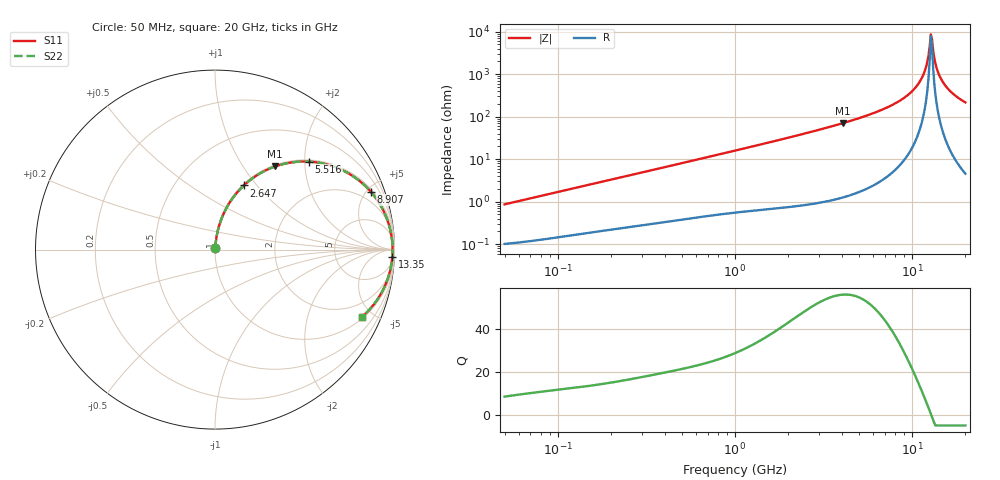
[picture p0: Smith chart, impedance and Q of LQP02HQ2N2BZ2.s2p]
!Murata Part Number: LQP02HQ2N2BZ2
!These Parameters are Measured in Series Mode Connection
!  o--[Z]--o
!Port1  Port2
!  o-------o
!Freq. Start=50[MHz] Stop=20[GHz], 401[Steps]
# Hz S RI R 50
!Freq.(Hz) S11(Real) S11(Imag) S21(Real) S21(Imag) S12(Real) S12(Imag) S22(Real) S22(Imag)
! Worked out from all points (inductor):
!   401 points, 50 MHz to 20 GHz, reference 50 ohm
!   read as one part in series: L = 2.71 nH near 51.52 MHz
!   highest Q = 56.1 at 4.088 GHz (marker M1), where L = 2.75 nH
!   self-resonance near 12.76 GHz
!   S11 on the Smith chart (normalised r, x): 50 MHz: 1.00, +0.02; 2.647 GHz: 1.02, +0.86; 5.516 GHz: 1.04, +2.10; 8.907 GHz: 1.18, +5.33; 13.35 GHz: 13, -46; 20 GHz: 1.09, -4.32
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5e7  0.00108 0.00854  0.9989 -0.00854  0.9989 -0.00854  0.00108 0.00854
1.364002e8  0.00225 0.0226  0.9977 -0.0226  0.9977 -0.0226  0.00225 0.0226
3.721004e8  0.00667 0.0594  0.9933 -0.0594  0.9933 -0.0594  0.00667 0.0594
1e9  0.0295 0.1526  0.9705 -0.1526  0.9705 -0.1526  0.0295 0.1526
2.647493e9  0.1608 0.3575  0.8392 -0.3575  0.8392 -0.3575  0.1608 0.3575
2.728004e9  0.1695 0.3654  0.8305 -0.3654  0.8305 -0.3654  0.1695 0.3654
4.087748e9  0.3353 0.4633  0.6647 -0.4633  0.6647 -0.4633  0.3353 0.4633
5.515528e9  0.5236 0.4901  0.4764 -0.4901  0.4764 -0.4901  0.5236 0.4901
7.442007e9  0.7464 0.4231  0.2536 -0.4231  0.2536 -0.4231  0.7464 0.4231
8.907419e9  0.8687 0.3215  0.1313 -0.3215  0.1313 -0.3215  0.8687 0.3215
1.019291e10  0.9387 0.2161  0.0613 -0.2161  0.0613 -0.2161  0.9387 0.2161
1.131968e10  0.9739 0.121  0.0261 -0.121  0.0261 -0.121  0.9739 0.121
1.201863e10  0.9851 0.0634  0.0149 -0.0634  0.0149 -0.0634  0.9851 0.0634
1.257102e10  0.989 0.0193  0.011 -0.0193  0.011 -0.0193  0.989 0.0193
1.276073e10  0.9894 0.00455  0.0106 -0.00455  0.0106 -0.00455  0.9894 0.00455
1.314879e10  0.9889 -0.025  0.0111 0.025  0.0111 0.025  0.9889 -0.025
1.334722e10  0.988 -0.0397  0.012 0.0397  0.012 0.0397  0.988 -0.0397
1.354865e10  0.9866 -0.0544  0.0134 0.0544  0.0134 0.0544  0.9866 -0.0544
1.396067e10  0.9826 -0.0836  0.0174 0.0836  0.0174 0.0836  0.9826 -0.0836
1.504638e10  0.9651 -0.1547  0.0349 0.1547  0.0349 0.1547  0.9651 -0.1547
1.696185e10  0.9168 -0.2592  0.0832 0.2592  0.0832 0.2592  0.9168 -0.2592
2e10  0.8185 -0.3751  0.1815 0.3751  0.1815 0.3751  0.8185 -0.3751
